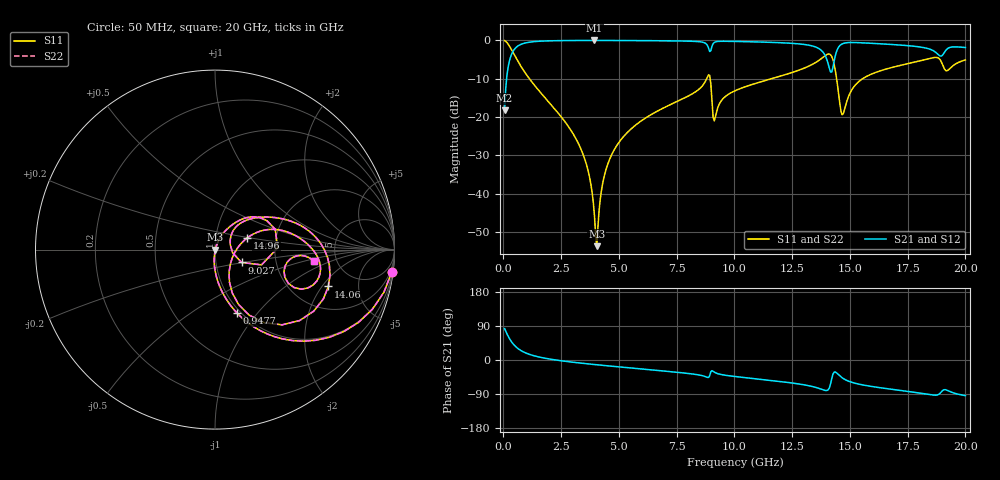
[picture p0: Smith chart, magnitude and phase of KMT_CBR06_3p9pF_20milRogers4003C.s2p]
! Data measured by Modelithics Inc. support@modelithics.com 813-866-6335
! KEMET CBR0603 3.9pF, Pad Width= 0.851mm, Pad Length= 0.64mm, Pad Gap= 0.62mm, 20mil Rogers 4003C substrate Data, January 2022
# hz S ma R 50
! 2 Port Network Data from SP1.SP block
! freq  magS11  angS11  magS21  angS21  magS12  angS12  magS22  angS22
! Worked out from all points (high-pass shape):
!   401 points, 50 MHz to 20 GHz, reference 50 ohm
!   highest |S21| = -0.02 dB at 3.94 GHz (marker M1); lowest = -18.2 dB at 50 MHz (marker M2)
!   |S21| within 3 dB of the highest: 400.9 MHz to 13.83 GHz (13.42 GHz wide, 189 % of centre); 14.42 GHz to 18.69 GHz (4.278 GHz wide, 25.8 % of centre)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
!   lowest |S11| = -53.7 dB at 4.04 GHz (marker M3), VSWR 1.00, Z = 50.2 + j0.00248 ohm
!   |S11| at or under -10 dB: 1.123 GHz to 8.798 GHz (7.675 GHz wide, 155 % of centre); 8.948 GHz to 11.61 GHz (2.661 GHz wide, 25.9 % of centre); 14.42 GHz to 15.55 GHz (1.129 GHz wide, 7.53 % of centre)
!   |S22| runs from -53.7 to -0.1 dB; largest |S21 - S12| = 0
!   S11 on the Smith chart (normalised r, x): 50 MHz: 1, -16; 947.8 MHz: 0.96, -0.79; 9.027 GHz: 1.33, -0.20; 14.06 GHz: 3.15, -2.31; 14.96 GHz: 1.42, +0.19; 20 GHz: 3.38, -0.62
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5e7  0.9924 -7.2  0.1226 82.8  0.1226 82.8  0.9924 -7.2
3.4925e8  0.7545 -42.1  0.6555 47.9  0.6555 47.9  0.7545 -42.1
9.4775e8  0.3747 -70.8  0.9261 19.0  0.9261 19.0  0.3747 -70.8
3.391625e9  0.0359 -95.6  0.9974 -8.5  0.9974 -8.5  0.0359 -95.6
3.74075e9  0.01568 -93.7  0.9978 -10.7  0.9978 -10.7  0.01568 -93.7
3.94025e9  0.005149 -79.4  0.9979 -12.0  0.9979 -12.0  0.005149 -79.4
4.04e9  0.002059 0.7  0.9979 -12.6  0.9979 -12.6  0.002059 0.7
4.33925e9  0.0157 68.0  0.9976 -14.4  0.9976 -14.4  0.0157 68.0
4.788125e9  0.03696 69.6  0.997 -17.0  0.997 -17.0  0.03696 69.6
6.73325e9  0.1224 60.8  0.9894 -27.9  0.9894 -27.9  0.1224 60.8
8.828e9  0.3308 29.2  0.8623 -45.9  0.8623 -45.9  0.3308 29.2
9.0275e9  0.1643 -25.8  0.8355 -28.3  0.8355 -28.3  0.1643 -25.8
9.177125e9  0.1018 33.5  0.9557 -33.7  0.9557 -33.7  0.1018 33.5
1.0025e10  0.22 44.9  0.9693 -43.6  0.9693 -43.6  0.22 44.9
1.336662e10  0.4851 16.9  0.8469 -69.9  0.8469 -69.9  0.4851 16.9
1.406488e10  0.6642 -18.0  0.4865 -78.2  0.4865 -78.2  0.6642 -18.0
1.431425e10  0.4913 -56.0  0.53 -32.3  0.53 -32.3  0.4913 -56.0
1.466338e10  0.1067 -26.2  0.8989 -46.9  0.8989 -46.9  0.1067 -26.2
1.496262e10  0.1921 20.1  0.9368 -56.4  0.9368 -56.4  0.1921 20.1
1.670825e10  0.434 11.9  0.8883 -76.5  0.8883 -76.5  0.434 11.9
1.895262e10  0.5286 -24.6  0.6234 -84.5  0.6234 -84.5  0.5286 -24.6
2e10  0.5556 -6.5  0.8071 -94.1  0.8071 -94.1  0.5556 -6.5
